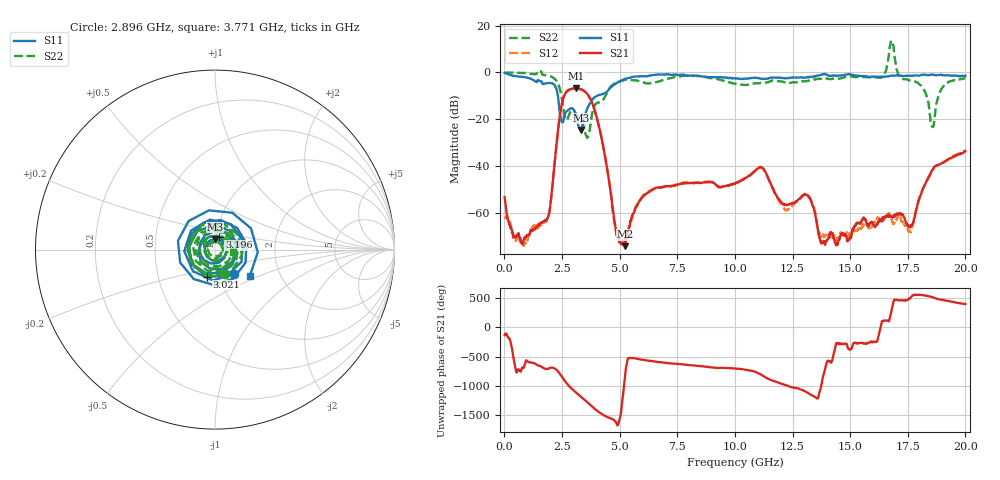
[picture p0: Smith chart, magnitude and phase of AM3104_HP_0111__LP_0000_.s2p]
!Created with skrf (http://scikit-rf.org).
# Hz S RI R 50.0
!freq ReS11 ImS11 ReS21 ImS21 ReS12 ImS12 ReS22 ImS22
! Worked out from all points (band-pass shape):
!   1601 points, 10 MHz to 20 GHz, reference 50 ohm
!   highest |S21| = -6.74 dB at 3.108 GHz (marker M1); lowest = -74.3 dB at 5.245 GHz (marker M2)
!   |S21| within 3 dB of the highest: 2.603 GHz to 3.637 GHz (1.034 GHz wide, 33.1 % of centre)
!   lowest |S11| = -24.7 dB at 3.321 GHz (marker M3), VSWR 1.12, Z = 49.7 + j5.83 ohm
!   |S11| at or under -10 dB: 2.322 GHz to 4.025 GHz (1.703 GHz wide, 53.7 % of centre)
!   |S22| runs from -28.0 to 13.7 dB; largest |S21 - S12| = 0.025
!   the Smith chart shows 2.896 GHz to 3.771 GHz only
!   S11 on the Smith chart (normalised r, x): 2.896 GHz: 1.19, -0.33; 3.021 GHz: 0.87, -0.27; 3.196 GHz: 1.04, +0.15; 3.771 GHz: 1.40, -0.44
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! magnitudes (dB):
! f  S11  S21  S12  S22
! 10 MHz  -0.2  -53.3  -61.6  0.0
! 759.6 MHz  -1.8  -72.8  -72.5  -0.3
! 1.847 GHz  -4.6  -62.9  -62.5  -1.2
! 2.471 GHz  -20.5  -14.5  -14.5  -9.7
! 2.896 GHz  -15.3  -7.1  -7.2  -16.5
! 3.021 GHz  -16.0  -6.9  -6.9  -16.4
! 3.108 GHz  -18.2  -6.7  -6.7  -17.8
! 3.196 GHz  -22.4  -6.8  -6.9  -18.8
! 3.321 GHz  -24.7  -7.2  -7.2  -19.9
! 3.346 GHz  -24.4  -7.3  -7.3  -20.4
! 3.771 GHz  -12.2  -12.2  -12.2  -20.0
! 4.845 GHz  -4.6  -67.4  -68.9  -4.4
! 5.245 GHz  -2.7  -74.3  -71.3  -3.1
! 6.682 GHz  -0.9  -49.3  -49.1  -3.9
! 10.01 GHz  -2.6  -47.7  -47.7  -4.8
! 11.14 GHz  -2.7  -40.6  -40.7  -4.5
! 13.34 GHz  -2.0  -56.1  -55.5  -3.3
! 13.82 GHz  -0.8  -72.3  -69.5  -2.6
! 16.68 GHz  -1.5  -61.6  -60.3  7.2
! 17.61 GHz  -1.4  -66.1  -68.2  -3.5
! 18.56 GHz  -0.9  -41.6  -41.9  -23.1
! 20 GHz  -1.4  -33.7  -33.5  -2.5
